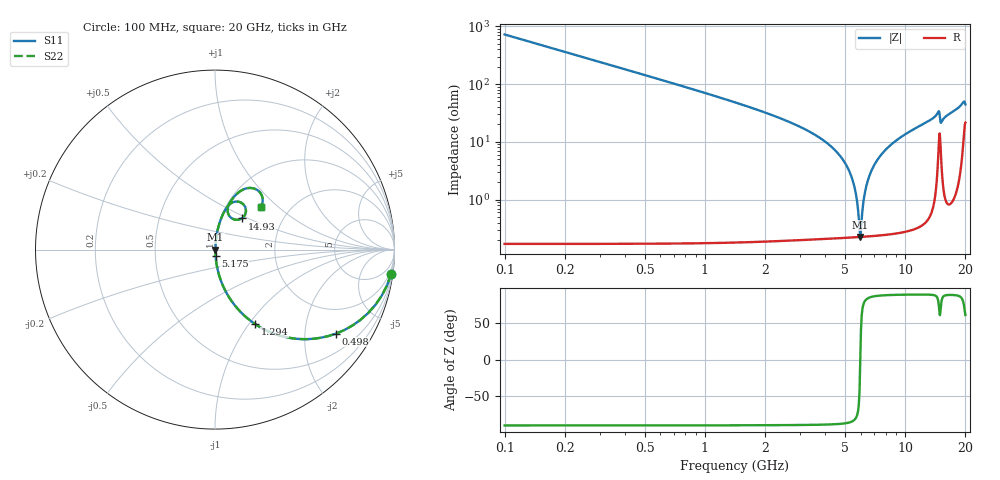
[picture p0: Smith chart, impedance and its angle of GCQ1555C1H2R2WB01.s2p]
!Murata Part Number: GCQ1555C1H2R2WB01
!These Parameters are Measured in Series Mode Connection
!Data Generated on Jan 08, 2026
!  o--ll--o
!Port1  Port2
!  o------o
!Operation Temp=25[degC], DC Bias Voltage=0[V]
!Freq. Start=100[MHz] Stop=20[GHz] 401[Steps]
# Hz S RI R 50
!Freq.(Hz) S11(Real) S11(Imag) S21(Real) S21(Imag) S12(Real) S12(Imag) S22(Real) S22(Imag)
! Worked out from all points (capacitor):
!   401 points, 100 MHz to 20 GHz, reference 50 ohm
!   read as one part in series: C = 2.2 pF near 199.5 MHz
!   lowest |Z| = 225 mohm at 5.971 GHz (marker M1)
!   series resonance near 5.972 GHz, so ESL is about 320 pH
!   S11 on the Smith chart (normalised r, x): 100 MHz: 1, -14; 498 MHz: 1.00, -2.89; 1.294 GHz: 1.00, -1.07; 5.175 GHz: 1.00, -0.07; 14.93 GHz: 1.26, +0.46; 20 GHz: 1.43, +0.78
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1e8  0.9812 -0.1357  0.0188 0.1357  0.0188 0.1357  0.9812 -0.1357
2.99e8  0.8533 -0.3535  0.1467 0.3535  0.1467 0.3535  0.8533 -0.3535
4.98e8  0.6752 -0.4677  0.3248 0.4677  0.3248 0.4677  0.6752 -0.4677
8.96e8  0.3841 -0.4853  0.6159 0.4853  0.6159 0.4853  0.3841 -0.4853
1.294e9  0.2219 -0.4139  0.7781 0.4139  0.7781 0.4139  0.2219 -0.4139
3.43325e9  0.0215 -0.138  0.9785 0.138  0.9785 0.138  0.0215 -0.138
4.478e9  0.0071 -0.0704  0.9929 0.0704  0.9929 0.0704  0.0071 -0.0704
5.1745e9  0.0034 -0.0349  0.9966 0.0349  0.9966 0.0349  0.0034 -0.0349
5.62225e9  0.00243 -0.0147  0.9976 0.0147  0.9976 0.0147  0.00243 -0.0147
5.9705e9  0.00224 -7.17e-05  0.9978 7.17e-05  0.9978 7.17e-05  0.00224 -7.17e-05
6.07e9  0.00227 0.00395  0.9977 -0.00395  0.9977 -0.00395  0.00227 0.00395
6.31875e9  0.00246 0.0137  0.9975 -0.0137  0.9975 -0.0137  0.00246 0.0137
6.7665e9  0.00325 0.0305  0.9968 -0.0305  0.9968 -0.0305  0.00325 0.0305
7.9605e9  0.00752 0.071  0.9925 -0.071  0.9925 -0.071  0.00752 0.071
1.005e10  0.0208 0.1329  0.9792 -0.1329  0.9792 -0.1329  0.0208 0.1329
1.338325e10  0.0588 0.2244  0.9412 -0.2244  0.9412 -0.2244  0.0588 0.2244
1.467675e10  0.1449 0.262  0.8551 -0.262  0.8551 -0.262  0.1449 0.262
1.49255e10  0.15 0.1736  0.85 -0.1736  0.85 -0.1736  0.15 0.1736
1.51245e10  0.0858 0.1805  0.9142 -0.1805  0.9142 -0.1805  0.0858 0.1805
1.67165e10  0.0931 0.2774  0.9069 -0.2774  0.9069 -0.2774  0.0931 0.2774
1.925375e10  0.1992 0.3434  0.8008 -0.3434  0.8008 -0.3434  0.1992 0.3434
2e10  0.2538 0.2388  0.7462 -0.2388  0.7462 -0.2388  0.2538 0.2388
